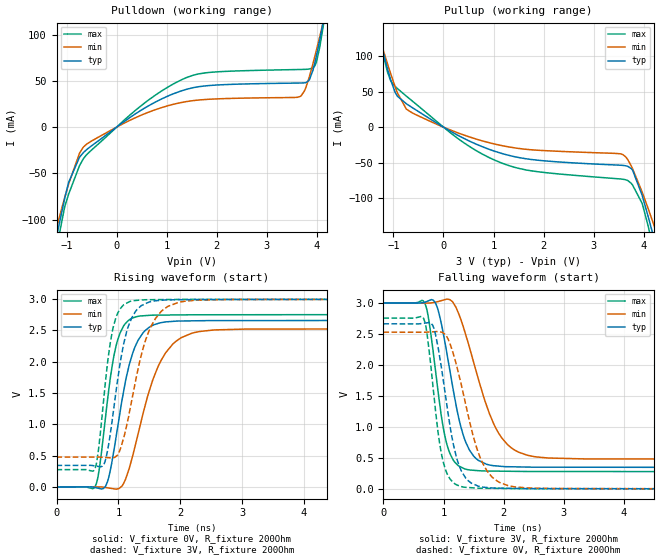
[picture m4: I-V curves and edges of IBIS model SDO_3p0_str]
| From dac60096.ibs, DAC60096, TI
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|   Model
[Model]   SDO_3p0_str
Model_type   Output
Polarity   Non-Inverting
Vmeas = 1.5
Vref = 0
Cref = 1pF
Rref = 100000
|   typ   min   max
C_comp   13.124pF   12.937pF   13.913pF
[Voltage Range]   3   2.999   3.001
[Temperature Range]   27   105   -40
[Pullup Reference]   3   2.999   3.001
[Pulldown Reference]   0   0   0
[Power Clamp Reference]   3   2.999   3.001
[GND Clamp Reference]   0   0   0
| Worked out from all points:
|   slope of the pulldown table from 0 to 0.45 V, typ, clamps not added: 26.6 ohm
|   slope of the pullup table from 0 to 0.45 V, typ, clamps not added: 26 ohm
|   falling waveform, V_fixture 3V, R_fixture 200Ohm: 20-80 % time 323ps typ, 503ps min, 235ps max; typ from 3 V to 0.345 V
|   rising waveform, V_fixture 0V, R_fixture 200Ohm: 20-80 % time 311ps typ, 458ps min, 225ps max; typ from 0 V to 2.66 V
|   rising waveform, V_fixture 3V, R_fixture 200Ohm: 20-80 % time 258ps typ, 363ps min, 193ps max; typ from 0.345 V to 3 V
|   falling waveform, V_fixture 0V, R_fixture 200Ohm: 20-80 % time 274ps typ, 401ps min, 206ps max; typ from 2.66 V to 0 V
[Pulldown]
|   Voltage   I(typ)   I(min)   I(max)
-3V       -641.7mA   -522.5mA   -768.4mA
-1.218V   -122.9mA   -112.1mA   -135.7mA
-957mV    -59.53mA   -61.2mA    -72.19mA
-660mV    -27.34mA   -21.36mA   -33.9mA
519mV     19.26mA    13.56mA    24.39mA
1.365V    40.36mA    27.33mA    52.81mA
3.669V    47.65mA    33.21mA    62.28mA
3.849V    50.99mA    54.21mA    62.79mA
3.957V    68.97mA    75.81mA    66.02mA
4.056V    93.79mA    97.44mA    85.9mA
4.155V    121.2mA    119.9mA    118.1mA
6V        685.9mA    569.8mA    836.3mA
[Pullup]
|   Voltage   I(typ)   I(min)   I(max)
-3V       652.9mA    545.4mA    798.9mA
-1.74V    263.9mA    235.8mA    303.3mA
-1.236V   114.4mA    116.1mA    114.2mA
-1.056V   66.9mA     75.75mA    65.5mA
-741mV    32.93mA    25.33mA    43.7mA
1.023V    -34.01mA   -23.86mA   -46.56mA
3.579V    -53.94mA   -38.62mA   -73.45mA
3.777V    -60.67mA   -58.66mA   -81.65mA
3.966V    -95.68mA   -91.17mA   -107.2mA
4.092V    -127mA     -115.6mA   -140.5mA
4.2V      -155.6mA   -137.5mA   -175.3mA
6V        -682.1mA   -553.3mA   -820mA
[Ramp]
R_load = 200
|   typ   min   max
dV/dt_r   1.59839/3.09679e-10   1.51747/4.58138e-10   1.65367/2.24694e-10
dV/dt_f   1.59301/3.22259e-10   1.51244/5.025e-10   1.63417/2.34577e-10
[Falling Waveform]
V_fixture = 3V
V_fixture_min = 2.999V
V_fixture_max = 3.001V
R_fixture = 200Ohm
C_fixture = 0F
|   Time   V(typ)   V(min)   V(max)
0s        3V         2.999V     3.001V
663.1ps   3.006V     2.999V     3.034V
740.6ps   3.032V     2.999V     2.806V
863ps     3.005V     3.011V     1.934V
1.063ns   2.149V     3.062V     697.2mV
1.351ns   804.1mV    2.543V     326.8mV
1.536ns   496.5mV    1.919V     301.4mV
1.842ns   377.4mV    1.034V     291.1mV
2.384ns   356.1mV    549.4mV    285.5mV
10ns      345mV      478.3mV    277.4mV
[Rising Waveform]
V_fixture = 0V
V_fixture_min = 0V
V_fixture_max = 0V
R_fixture = 200Ohm
C_fixture = 0F
|   Time   V(typ)   V(min)   V(max)
0s        -177.8nV   201.5pV    -420.3nV
607.4ps   -4.944mV   1.024mV    -15.28mV
677.1ps   -19.91mV   1.142mV    203.1mV
792.1ps   11.81mV    -7.869mV   1.117V
985.2ps   939.2mV    -30.09mV   2.339V
1.132ns   1.771V     170.9mV    2.629V
1.279ns   2.261V     687.8mV    2.716V
1.691ns   2.624V     2.023V     2.745V
2.247ns   2.654V     2.47V      2.75V
10ns      2.664V     2.529V     2.756V
[Rising Waveform]
V_fixture = 3V
V_fixture_min = 2.999V
V_fixture_max = 3.001V
R_fixture = 200Ohm
C_fixture = 0F
|   Time   V(typ)   V(min)   V(max)
0s        344.7mV    477.5mV    277.4mV
621ps     337mV      478.3mV    292.3mV
768.2ps   368.2mV    472.6mV    1.458V
921.9ps   1.231V     469.2mV    2.573V
1.04ns    2.052V     632.2mV    2.859V
1.184ns   2.626V     1.223V     2.962V
1.361ns   2.889V     2.075V     2.985V
1.53ns    2.963V     2.571V     2.991V
2.016ns   2.991V     2.957V     2.995V
10ns      3V         2.999V     3.001V
[Falling Waveform]
|Gnd
V_fixture = 0V
V_fixture_min = 0V
V_fixture_max = 0V
R_fixture = 200Ohm
C_fixture = 0F
|   Time   V(typ)   V(min)   V(max)
0s        2.664V     2.529V     2.756V
652.5ps   2.671V     2.529V     2.775V
717ps     2.68V      2.53V      2.555V
818.9ps   2.641V     2.536V     1.704V
997.9ps   1.738V     2.513V     426.1mV
1.162ns   726.1mV    2.182V     105.6mV
1.279ns   333.3mV    1.75V      45.79mV
1.659ns   32.64mV    400.1mV    14.56mV
2.125ns   13.33mV    46.22mV    10.24mV
10ns      259.2uV    808.3uV    51.03uV
